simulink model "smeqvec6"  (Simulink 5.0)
settings: Solver=ode45  StartTime=0.0  StopTime=100  MaxStep=.05  RelTol=1e-4  AbsTol=1e-4
InitFcn:
  | smvecdef6
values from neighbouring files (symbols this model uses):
  Bm = 0.10    (= 0.1)    [IMabc2.m]    (also in imabcparam.m = 0.01; IMabcrun0.m = 0.01; IMabcrun1.m = 0.001; IMcur0.m = 1e-06)
  H = 0.60    (= 0.6)    [IMabc2.m]    (also in IMcur0.m = 0.3; imdef0vec.m = 0.3; imdef1vec.m = 0.3; imdef2vec.m = 0.3)
  n0 = 0.98    [imdef0vec.m]    (also in imdef1vec.m = 0.978; imdef2vec.m; imdefrotflux.m; imdefSIvec1.m = 0.95)
  Ra = .95    (= 0.95)    [altwdgs.m]    (also in Ccurverun.m = 0.018)
  wo = 2*pi*freq0    [calc0.m]    (also in IMabc2.m = 376.991118431; imabcparam.m = 376.991118431; IMabcrun0.m = 376.991118431; IMabcrun1.m = 376.991118431)
undefined symbols (not defined in the file or in its folder): delta0, fa0, fk0, L_1, phif0, Rf, Rkd, Rkq, vf0
libraries: simulink x3

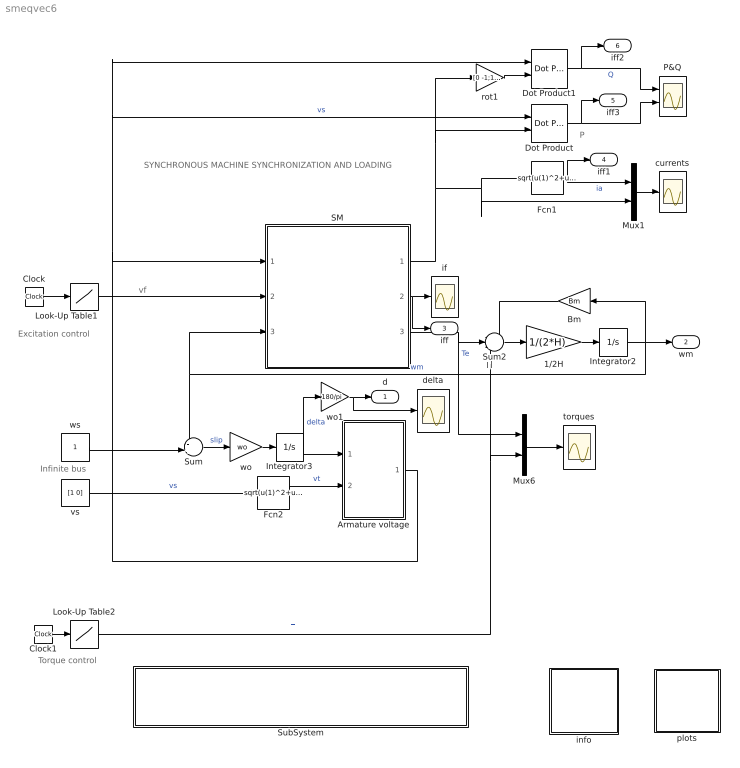
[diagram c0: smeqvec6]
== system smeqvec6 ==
  note: Tl
  note: P
  note: Excitation control
  note: Torque control
  note: SYNCHRONOUS MACHINE SYNCHRONIZATION AND LOADING
  note: vf
  note: Infinite bus
  1/2H : Gain  Gain=1/(2*H)
  Armature voltage : Subsystem
  Bm : Gain  Orientation=left  Gain=Bm
  Clock : Clock
  Clock1 : Clock
  Dot Product : simulink/Math Operations/Dot Product
  Dot Product1 : simulink/Math Operations/Dot Product
  Fcn1 : Fcn  Expr=sqrt(u(1)^2+u(2)^2)
  Fcn2 : Fcn  Expr=sqrt(u(1)^2+u(2)^2)
  Integrator2 : Integrator  InitialCondition=n0
  Integrator3 : Integrator  InitialCondition=delta0
  Look-Up Table1 : Lookup  InputValues="[0  20  30 40 60 80]"  OutputValues="[vf0 vf0 4*vf0  4*vf0 0.7*vf0 0.7*vf0]"
  Look-Up Table2 : Lookup  InputValues="[0  10  15 100]"  OutputValues=[0 0 -.75 -.75]
  Mux1 : Mux  Inputs=2
  Mux6 : Mux  Inputs=2
  P&Q : Scope  NumInputPorts=2
  SM : Subsystem
  SubSystem : Subsystem
  Sum : Sum  Inputs=-+|
  Sum2 : Sum  Inputs=-+-
  currents : Scope
  delta : Scope
  if : Scope
  info : Subsystem
  plots : Subsystem
  rot1 : Gain  Gain=[0 -1;1 0]  Multiplication=Matrix(K*u)
  torques : Scope
  vs : Constant  Value=[1 0]
  wo : Gain  Gain=wo
  wo1 : Gain  Gain=180/pi
  ws : Constant
  d : Outport
  wm : Outport  Port=2
  iff : Outport  Port=3
  iff1 : Outport  Port=4
  iff3 : Outport  Port=5
  iff2 : Outport  Port=6
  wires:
  1/2H/1 -> Integrator2/1
  Sum2/1 -> 1/2H/1
  Bm/1 -> Sum2/1
  SM/3(Te) -> Mux6/1, Sum2/2  "Te"
  Mux6/1 -> torques/1
  SM/1(ia) -> Dot Product/2, rot1/1, Fcn1/1, Mux1/2
  SM/2(if) -> if/1, iff/1
  Integrator2/1 -> Bm/1, Sum/1, SM/3(wm), wm/1  "wm"
  ws/1 -> Sum/2
  Sum/1 -> wo/1  "slip"
  Armature voltage/1(vs) -> SM/1(vs), Dot Product/1, Dot Product1/1  "vs"
  wo/1 -> Integrator3/1
  Integrator3/1 -> Armature voltage/1(delta), wo1/1  "delta"
  Dot Product/1 -> P&Q/2, iff3/1
  Dot Product1/1 -> P&Q/1, iff2/1  "Q"
  rot1/1 -> Dot Product1/2
  Clock/1 -> Look-Up Table1/1
  Look-Up Table1/1 -> SM/2(vf)
  Clock1/1 -> Look-Up Table2/1
  Fcn1/1 -> iff1/1, Mux1/1  "ia"
  Look-Up Table2/1 -> Sum2/3, Mux6/2  "Tl"
  Mux1/1 -> currents/1
  wo1/1 -> delta/1, d/1
  Fcn2/1 -> Armature voltage/2(Vt)  "vt"
  vs/1 -> Fcn2/1  "vs"

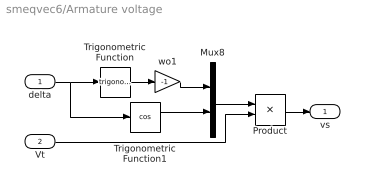
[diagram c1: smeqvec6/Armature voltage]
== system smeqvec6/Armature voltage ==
  delta : Inport
  Vt : Inport  Port=2
  Mux8 : Mux  Inputs=2
  Product : Product
  Trigonometric Function : Trigonometry
  Trigonometric Function1 : Trigonometry  Operator=cos
  wo1 : Gain  Gain=-1
  vs : Outport
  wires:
  delta/1 -> Trigonometric Function/1, Trigonometric Function1/1
  Trigonometric Function/1 -> wo1/1
  Mux8/1 -> Product/1
  wo1/1 -> Mux8/1
  Trigonometric Function1/1 -> Mux8/2
  Product/1 -> vs/1
  Vt/1 -> Product/2

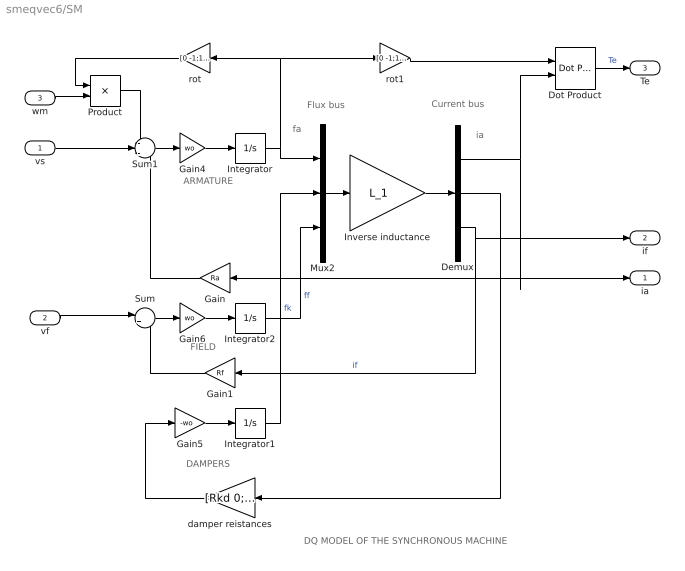
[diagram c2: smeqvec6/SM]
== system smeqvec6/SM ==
  note: DAMPERS
  note: ARMATURE
  note: fa
  note: ia
  note: FIELD
  note: DQ MODEL OF THE SYNCHRONOUS MACHINE
  note: Flux bus
  note: Current bus
  vs : Inport
  vf : Inport  Port=2
  wm : Inport  Port=3
  Demux : Demux  Outputs=3
  Dot Product : simulink/Math Operations/Dot Product
  Gain : Gain  Orientation=left  Gain=Ra
  Gain1 : Gain  Orientation=left  Gain=Rf
  Gain4 : Gain  Gain=wo
  Gain5 : Gain  Gain=-wo
  Gain6 : Gain  Gain=wo
  Integrator : Integrator  InitialCondition=fa0
  Integrator1 : Integrator  InitialCondition=fk0
  Integrator2 : Integrator  InitialCondition=phif0
  Inverse inductance : Gain  Gain=L_1  Multiplication=Matrix(K*u)
  Mux2 : Mux  Inputs=3
  Product : Product
  Sum : Sum  Inputs=|+-
  Sum1 : Sum  Inputs=-+-
  damper reistances : Gain  Orientation=left  Gain=[Rkd 0;0 Rkq]  Multiplication=Matrix(K*u)
  rot : Gain  Orientation=left  Gain=[0 -1;1 0]  Multiplication=Matrix(K*u)
  rot1 : Gain  Gain=[0 -1;1 0]  Multiplication=Matrix(K*u)
  ia : Outport
  if : Outport  Port=2
  Te : Outport  Port=3
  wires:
  Product/1 -> Sum1/1
  rot/1 -> Product/1
  wm/1 -> Product/2
  Gain5/1 -> Integrator1/1
  damper reistances/1 -> Gain5/1
  Integrator/1 -> Mux2/1, rot/1, rot1/1
  Sum1/1 -> Gain4/1
  Gain4/1 -> Integrator/1
  vs/1 -> Sum1/2
  Gain/1 -> Sum1/3
  Gain6/1 -> Integrator2/1
  Sum/1 -> Gain6/1
  vf/1 -> Sum/1
  Gain1/1 -> Sum/2
  rot1/1 -> Dot Product/1
  Demux/1 -> Gain/1, ia/1, Dot Product/2
  Dot Product/1 -> Te/1  "Te"
  Mux2/1 -> Inverse inductance/1
  Inverse inductance/1 -> Demux/1
  Integrator1/1 -> Mux2/2  "fk"
  Integrator2/1 -> Mux2/3  "ff"
  Demux/2 -> damper reistances/1
  Demux/3 -> if/1, Gain1/1  "if"

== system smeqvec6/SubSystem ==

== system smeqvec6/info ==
  note: The synchronous machine is running at no load at or close to synchronous speed when connected to an infinite bus. The transients occurring during the synchronization process will depend on the initial state defined by the excitation no-load voltage Ef, the speed, and the phase (torque) angle. Once synchronized, the machine is slowly loaded: first the real power absorbed P is ajusted by ramping the input torque (negatively for generator operation and positively for motor operation); then the reactive power absorbed Q is adjusted by controlling the voltage vf applied to the field (increasing the field and then weakening it in order to operate in over- and under-excited modes). Because of the slow ramping of these inputs, the machine system is in quasi equilibrium and is essentially in steady state at every loading condition. As a consequence, steady-state characteristics of the synchronous machine can be obtained such as V_curves. Note that the system becomes unstable if the field excitation reaches a specific low threshold that depends on the established active load P.
  note: SYNCHRONOUS MACHINE AGAINST AN INFINITE BUS
  note: SYNCHRONIZATION AND LOADING

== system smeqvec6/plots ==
